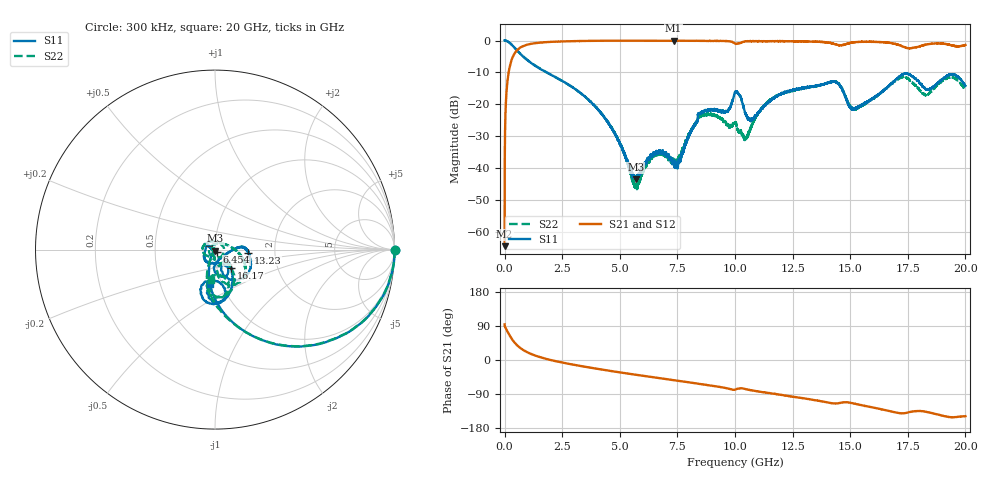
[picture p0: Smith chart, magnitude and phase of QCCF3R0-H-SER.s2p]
!QCCF3R0
!Johanson Technology Inc.
!www.johansontechnology.com
!Test Board Conditions:
!Substrate Type  RO4350B
!Substrate Thickness  10 mil
!Substrate Dk  3.66
!TL Type: GCPW
!TL Trace Width  21 mil
!TL Gap  20 mil
!Electrode orientation  Horizontal
!DUT TOPOLOGY	SERIES
!Mounting Pad LxW  16x21 mil
# MHz S  dB  R 50
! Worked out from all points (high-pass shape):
!   20001 points, 300 kHz to 20 GHz, reference 50 ohm
!   highest |S21| = -0.03 dB at 7.332 GHz (marker M1); lowest = -64.5 dB at 300 kHz (marker M2)
!   |S21| within 3 dB of the highest: 542.1 MHz to end of sweep
!   lowest |S11| = -43.6 dB at 5.688 GHz (marker M3), VSWR 1.01, Z = 50.1 - j0.656 ohm
!   |S11| at or under -10 dB: 1.815773 GHz to 1.816473 GHz (700 kHz wide, 0.0385 % of centre); 1.818 GHz to end of sweep
!   |S22| runs from -46.7 to 0.0 dB; largest |S21 - S12| = 0.02
!   S11 on the Smith chart (normalised r, x): 300 kHz: open; 6.454 GHz: 1.02, -0.03; 13.23 GHz: 1.45, -0.05; 16.17 GHz: 1.17, -0.25; 20 GHz: 0.88, -0.35
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0.3  0.03 -0.2  -64.53 93.9  -64.88 96.8  0.02 0.0
123.298  -0.22 -14.5  -12.77 75.3  -12.80 75.3  -0.23 -14.6
413.294  -2.09 -42.0  -4.27 47.5  -4.26 47.6  -2.12 -41.9
1278.281  -7.65 -76.6  -0.87 12.8  -0.85 12.7  -7.61 -76.9
3334.25  -16.68 -103.3  -0.13 -16.2  -0.13 -16.1  -16.71 -108.0
4707.229  -28.31 -120.6  -0.05 -29.9  -0.04 -29.9  -28.13 -115.8
5688.215  -43.58 -80.9  -0.06 -38.9  -0.06 -38.9  -45.74 179.3
6454.203  -35.62 -51.8  -0.06 -45.5  -0.06 -45.5  -36.03 134.0
6667.2  -35.34 -58.3  -0.06 -47.4  -0.06 -47.4  -35.74 137.2
7332.19  -38.45 -104.2  -0.03 -53.1  -0.04 -53.1  -38.12 -179.1
8495.173  -22.90 -145.7  -0.08 -63.3  -0.10 -63.3  -23.87 -158.0
9623.156  -22.18 -81.3  -0.16 -74.4  -0.18 -74.2  -26.24 110.4
10000.15  -16.23 -63.0  -0.92 -78.4  -0.92 -78.1  -25.74 -34.0
10726.14  -24.60 -43.8  -0.20 -80.0  -0.14 -80.1  -26.62 47.8
11589.13  -18.67 3.2  -0.21 -88.1  -0.18 -88.5  -18.48 -4.0
13234.1  -14.62 -5.3  -0.31 -103.6  -0.32 -103.4  -14.62 -26.2
13334.1  -14.53 -6.3  -0.34 -104.5  -0.36 -104.6  -14.54 -27.5
14415.08  -13.19 -47.3  -1.29 -114.4  -1.31 -114.2  -13.02 -61.4
15123.07  -21.36 -54.9  -0.56 -114.3  -0.58 -114.6  -21.58 -65.6
16169.06  -17.17 -48.6  -0.43 -127.6  -0.34 -127.4  -17.40 -47.9
16667.05  -14.32 -59.5  -0.68 -134.1  -0.65 -134.8  -14.25 -55.8
20000  -14.29 -98.7  -1.39 -148.5  -1.25 -147.9  -15.35 -97.7
